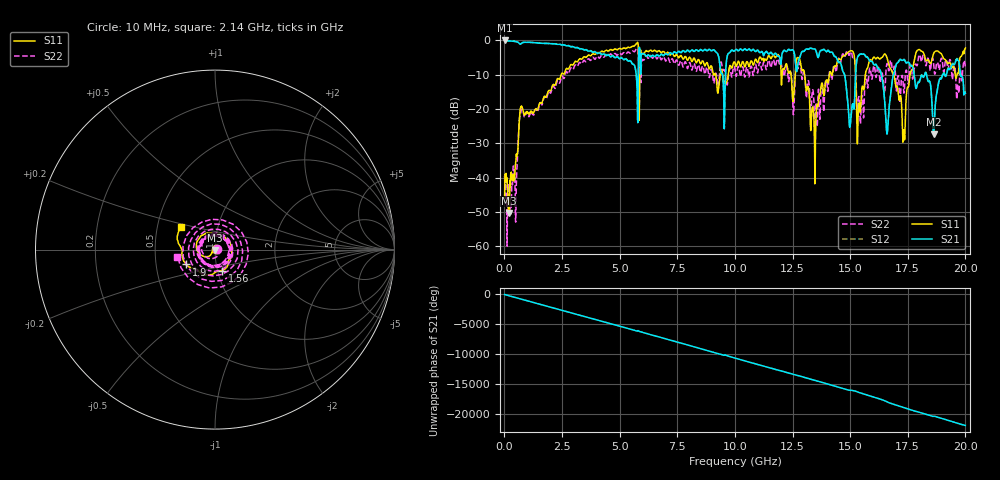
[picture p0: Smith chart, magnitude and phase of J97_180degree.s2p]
!Keysight Technologies,N5222A,MY51421036,A.10.65.16
!Date: Friday, March 31, 2023 14:32:30
!Correction: S11(Full 2 Port(1,2))
!S21(Full 2 Port(1,2))
!S12(Full 2 Port(1,2))
!S22(Full 2 Port(1,2))
!S2P File: Measurements: S11, S21, S12, S22:
# Hz S  dB  R 50
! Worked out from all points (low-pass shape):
!   2000 points, 10 MHz to 20 GHz, reference 50 ohm
!   highest |S21| = -0.05 dB at 10 MHz (marker M1); lowest = -27.3 dB at 18.62 GHz (marker M2)
!   |S21| within 3 dB of the highest: start of sweep to 3.607 GHz; 10.15 GHz to 10.7 GHz (550.6 MHz wide, 5.28 % of centre)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
!   lowest |S11| = -50.3 dB at 180 MHz (marker M3), VSWR 1.01, Z = 49.8 - j0.235 ohm
!   |S11| at or under -10 dB: start of sweep to 2.465 GHz; 13.03 GHz to 14.1 GHz (1.072 GHz wide, 7.9 % of centre); 16.89 GHz to 17.6 GHz (707.6 MHz wide, 4.1 % of centre)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
!   |S22| runs from -60.0 to -2.3 dB; largest |S21 - S12| = 0.026
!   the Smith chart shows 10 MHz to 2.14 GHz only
!   S11 on the Smith chart (normalised r, x): 10 MHz: 1.01, +0.01; 1.56 GHz: 1.05, -0.25; 1.9 GHz: 0.71, -0.12; 2.14 GHz: 0.66, +0.17
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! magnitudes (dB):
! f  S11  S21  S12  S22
! 10 MHz  -45.8  0.0  -0.1  -39.5
! 180 MHz  -50.3  -0.2  -0.2  -42.1
! 730 MHz  -19.3  -0.9  -0.9  -20.4
! 1.56 GHz  -18.1  -0.9  -0.8  -18.2
! 1.9 GHz  -14.9  -1.0  -0.9  -15.1
! 2.14 GHz  -12.9  -1.1  -1.0  -13.4
! 3.35 GHz  -5.5  -2.5  -2.4  -6.9
! 6.68 GHz  -3.1  -4.6  -4.5  -4.8
! 9.5 GHz  -12.3  -12.9  -12.8  -8.7
! 10.01 GHz  -6.8  -2.9  -2.9  -8.8
! 12.76 GHz  -5.1  -6.0  -6.0  -7.6
! 13.34 GHz  -20.7  -2.4  -2.4  -16.1
! 14.53 GHz  -5.5  -6.4  -6.4  -5.6
! 15.01 GHz  -3.1  -24.3  -24.3  -3.5
! 15.37 GHz  -18.9  -4.5  -4.4  -16.5
! 15.68 GHz  -9.2  -4.7  -4.7  -10.2
! 16.67 GHz  -6.9  -21.5  -21.4  -8.9
! 17.32 GHz  -26.1  -5.7  -5.5  -14.6
! 17.88 GHz  -3.2  -13.9  -13.5  -7.3
! 18.62 GHz  -3.8  -27.3  -27.2  -6.6
! 19.61 GHz  -10.8  -5.7  -5.5  -15.7
! 20 GHz  -2.3  -15.4  -15.1  -7.9
